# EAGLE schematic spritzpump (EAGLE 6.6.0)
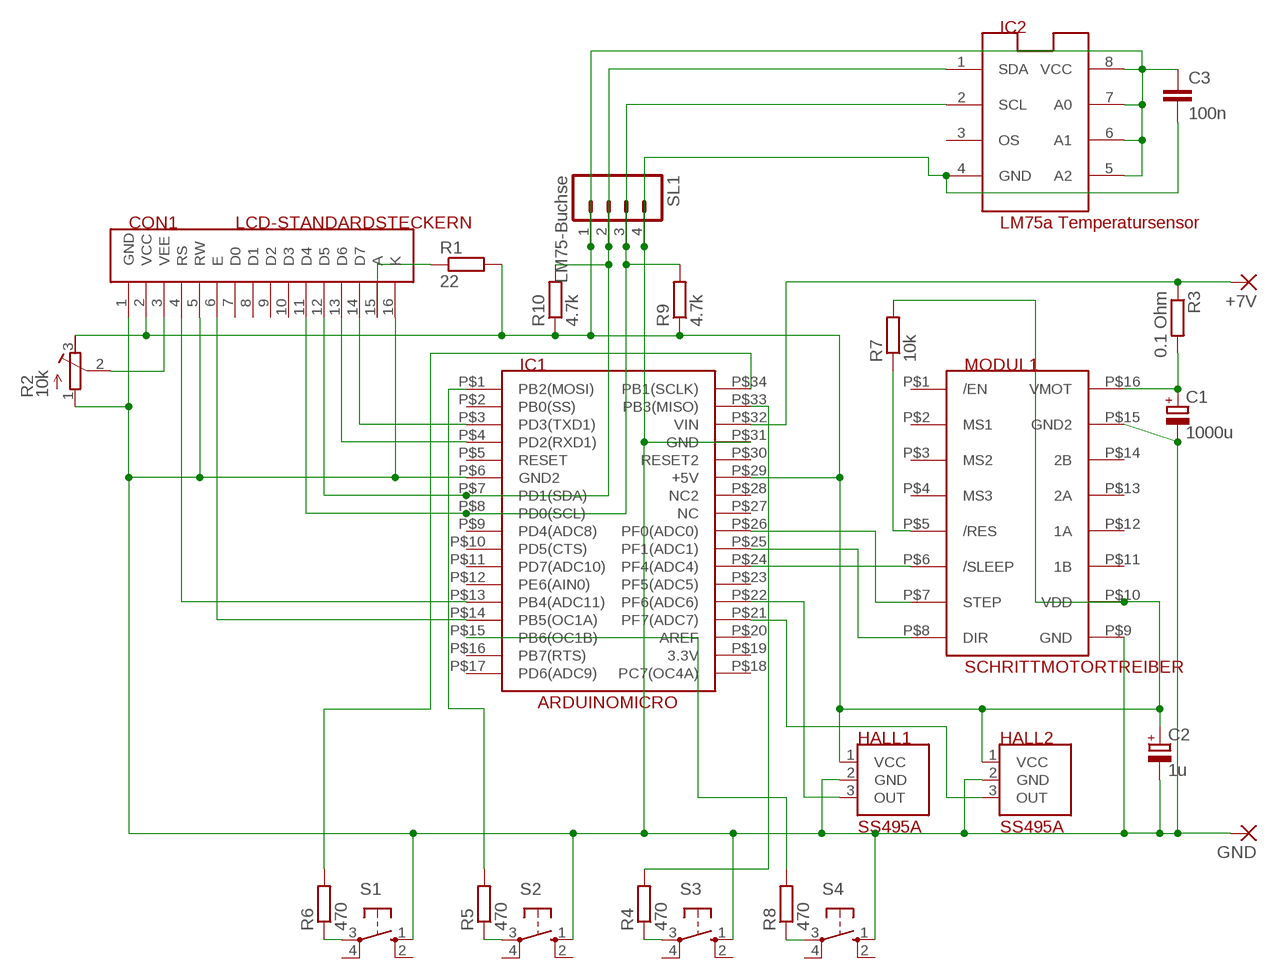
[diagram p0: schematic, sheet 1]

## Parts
+7V  1,6/0,8  [1,6/0,8]
C1  1000u  CPOL-EUE7.5-16  [E7,5-16]
C2  1u  CPOL-EUE2.5-5  [E2,5-5]
C3  100n  C-EUC1206  [C1206]
CON1  LCD-STANDARDSTECKERN  [STECKER16]
GND  1,6/0,8  [1,6/0,8]
HALL1  SS495A  [SS495A]
HALL2  SS495A  [SS495A]
IC1  ARDUINOMICRO  [ARDUINOMICRO]
IC2  LM75a Temperatursensor  LM75_ICN  [SO8_LM75]
MODUL1  SCHRITTMOTORTREIBER  [SCHRITTMOTORTREIBER]
R1  22  R-EU_0204/7  [0204/7]
R2  10k  R-TRIMM4G/J  [RTRIM4G/J]
R3  0.1 Ohm  R-EU_0204/7  [0204/7]
R4  470  R-EU_0204/7  [0204/7]
R5  470  R-EU_0204/7  [0204/7]
R6  470  R-EU_0204/7  [0204/7]
R7  10k  R-EU_0204/7  [0204/7]
R8  470  R-EU_0204/7  [0204/7]
R9  4.7k  R-EU_0204/7  [0204/7]
R10  4.7k  R-EU_0204/7  [0204/7]
S1  10-XX  [B3F-10XX]
S2  10-XX  [B3F-10XX]
S3  10-XX  [B3F-10XX]
S4  10-XX  [B3F-10XX]
SL1  LM75-Buchse  M04  [04P]

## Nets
GND: C1.- C2.- C3.2 CON1.1(GND) CON1.5(RW) CON1.16(K) GND.1(P) HALL1.2(GND) HALL2.2(GND) IC1.P$6(GND2) IC1.P$31(GND) IC2.4(GND) MODUL1.P$9(GND) MODUL1.P$15(GND2) R2.1(E) S1.1(S) S2.1(S) S3.1(S) S4.1(S) SL1.4
N$1: IC1.P$26(PF0(ADC0)) MODUL1.P$7(STEP)
N$2: R6.1 S1.3(P)
N$3: CON1.11(D4) IC1.P$8(PD0(SCL)) IC2.2(SCL) R9.2 SL1.3
N$4: CON1.12(D5) IC1.P$7(PD1(SDA)) IC2.1(SDA) R10.2 SL1.2
N$5: CON1.13(D6) IC1.P$4(PD2(RXD1))
N$6: CON1.14(D7) IC1.P$3(PD3(TXD1))
N$7: CON1.4(RS) IC1.P$13(PB4(ADC11))
N$8: CON1.6(E) IC1.P$14(PB5(OC1A))
N$9: CON1.15(A) R1.1
N$10: CON1.3(VEE) R2.2(S)
N$11: IC1.P$25(PF1(ADC1)) MODUL1.P$8(DIR)
N$12: MODUL1.P$5(/RES) R7.1
N$13: R5.1 S2.3(P)
N$14: R4.1 S3.3(P)
N$15: IC1.P$34(PB1(SCLK)) R6.2
N$16: IC1.P$1(PB2(MOSI)) R5.2
N$17: IC1.P$33(PB3(MISO)) R4.2
N$18: HALL1.3(OUT) IC1.P$22(PF6(ADC6))
N$19: HALL2.3(OUT) IC1.P$21(PF7(ADC7))
N$20: IC1.P$15(PB6(OC1B)) R8.2
N$21: IC1.P$24(PF4(ADC4)) MODUL1.P$6(/SLEEP)
N$22: R8.1 S4.3(P)
VCC: C2.+ C3.1 CON1.2(VCC) HALL1.1(VCC) HALL2.1(VCC) IC1.P$29(+5V) IC2.5(A2) IC2.6(A1) IC2.7(A0) IC2.8(VCC) MODUL1.P$10(VDD) R1.2 R2.3(A) R7.2 R9.1 R10.1 SL1.1
VIN: +7V.1(P) IC1.P$32(VIN) R3.1
VMOT: C1.+ MODUL1.P$16(VMOT) R3.2
Unconnected: CON1.7(D0) CON1.8(D1) CON1.9(D2) CON1.10(D3) IC1.P$2(PB0(SS)) IC1.P$5(RESET) IC1.P$9(PD4(ADC8)) IC1.P$10(PD5(CTS)) IC1.P$11(PD7(ADC10)) IC1.P$12(PE6(AIN0)) IC1.P$16(PB7(RTS)) IC1.P$17(PD6(ADC9)) IC1.P$18(PC7(OC4A)) IC1.P$19(3.3V) IC1.P$20(AREF) IC1.P$23(PF5(ADC5)) IC1.P$27(NC) IC1.P$28(NC2) IC1.P$30(RESET2) IC2.3(OS) MODUL1.P$1(/EN) MODUL1.P$2(MS1) MODUL1.P$3(MS2) MODUL1.P$4(MS3) MODUL1.P$11(1B) MODUL1.P$12(1A) MODUL1.P$13(2A) MODUL1.P$14(2B) S1.2(S1) S1.4(P1) S2.2(S1) S2.4(P1) S3.2(S1) S3.4(P1) S4.2(S1) S4.4(P1)

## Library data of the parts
+7V GND = wirepad:1,6/0,8: THROUGH-HOLE PAD
C1 C2 = rcl:CPOL-EU: POLARIZED CAPACITOR, European symbol
C3 = rcl:C-EU: CAPACITOR, European symbol
CON1 = 6_stecker:LCD-STANDARDSTECKER: Standard-Stecker fuer die meisten LCD-Module
HALL1 HALL2 = hallsensor:SS495A
IC1 = arduinomicro:ARDUINOMICRO
IC2 = lm75:LM75_IC: Temperatursensor
MODUL1 = arduino:SCHRITTMOTORTREIBER
R1 R3-R10 = resistor:R-EU_: RESISTOR, European symbol
R2 = resistor:R-TRIMM: Trimm resistor
S1-S4 = switch-omron:10-XX: OMRON SWITCH; MPN: B3F-1000; OC_FARNELL: 176432; OC_NEWARK: 36M3542
SL1 = con-amp-quick:M04: AMP QUICK CONNECTOR; OC_FARNELL: unknown; OC_NEWARK: unknown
